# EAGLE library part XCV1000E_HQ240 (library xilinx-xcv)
xcv1000e_hq240 edit this description Auto generated by make-symbol-device-package-bsdl.ulp Rev. 26 Source: xcv1000e_hq240.bsd
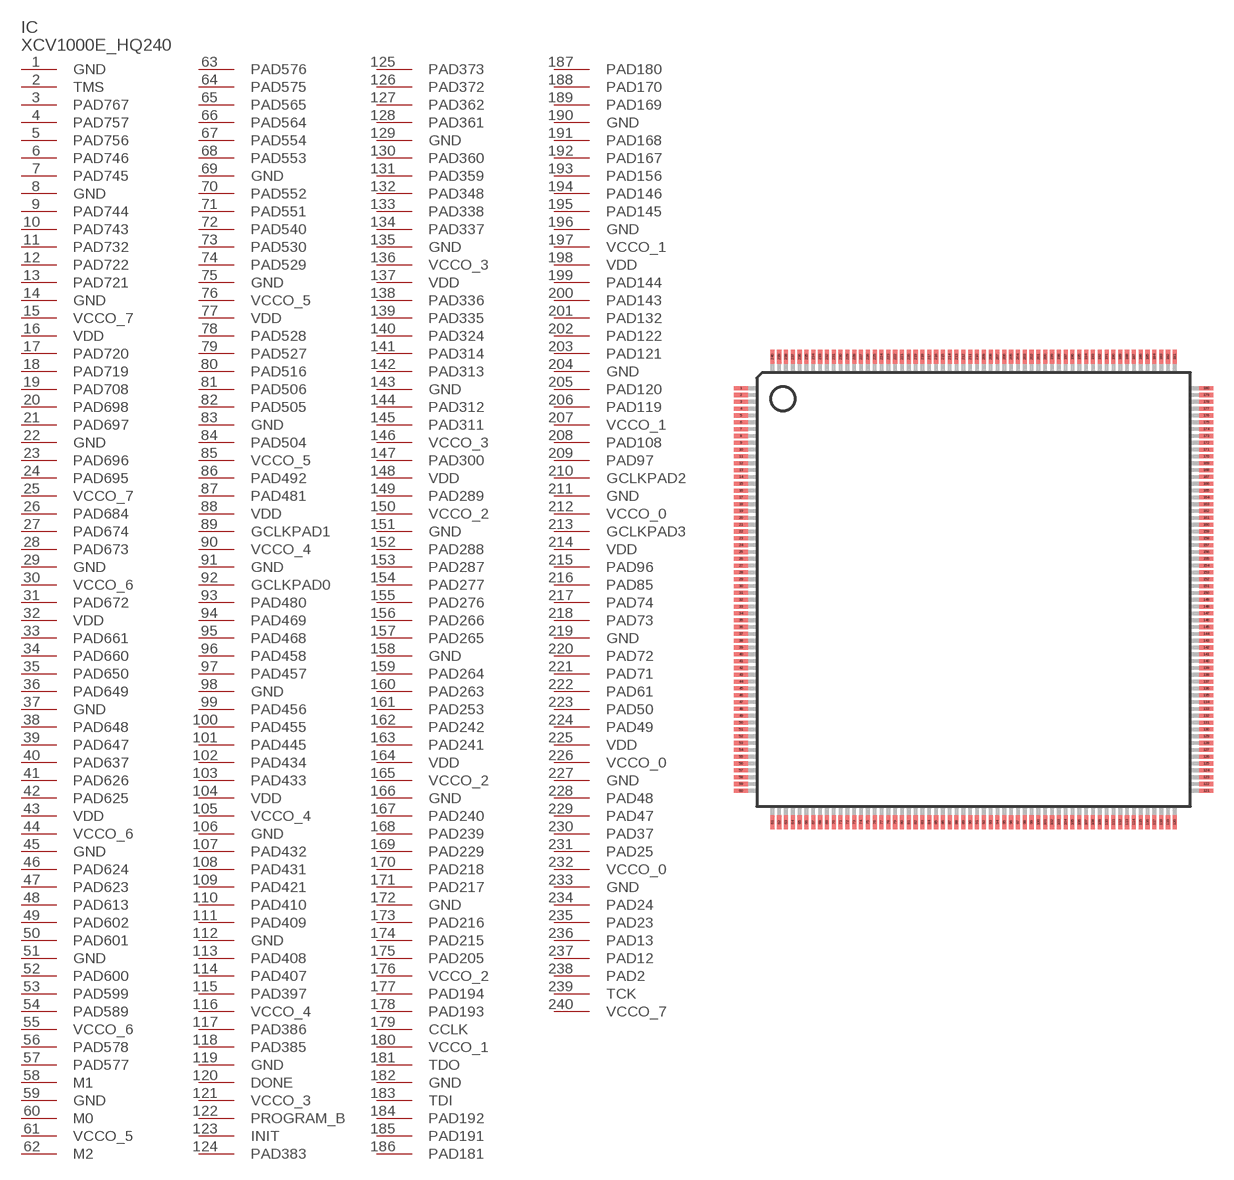
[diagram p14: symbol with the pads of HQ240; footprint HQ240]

Designator prefix IC

## XCV1000E_HQ240 (OC_FARNELL: unknown; OC_NEWARK: unknown)  [HQ240]
1  GND  pwr
2  TMS  in
3  PAD767
4  PAD757
5  PAD756
6  PAD746
7  PAD745
8  GND  pwr
9  PAD744
10  PAD743
11  PAD732
12  PAD722
13  PAD721
14  GND  pwr
15  VCCO_7  pwr
16  VDD  pwr
17  PAD720
18  PAD719
19  PAD708
20  PAD698
21  PAD697
22  GND  pwr
23  PAD696
24  PAD695
25  VCCO_7  pwr
26  PAD684
27  PAD674
28  PAD673
29  GND  pwr
30  VCCO_6  pwr
31  PAD672
32  VDD  pwr
33  PAD661
34  PAD660
35  PAD650
36  PAD649
37  GND  pwr
38  PAD648
39  PAD647
40  PAD637
41  PAD626
42  PAD625
43  VDD  pwr
44  VCCO_6  pwr
45  GND  pwr
46  PAD624
47  PAD623
48  PAD613
49  PAD602
50  PAD601
51  GND  pwr
52  PAD600
53  PAD599
54  PAD589
55  VCCO_6  pwr
56  PAD578
57  PAD577
58  M1  in
59  GND  pwr
60  M0  in
61  VCCO_5  pwr
62  M2  in
63  PAD576
64  PAD575
65  PAD565
66  PAD564
67  PAD554
68  PAD553
69  GND  pwr
70  PAD552
71  PAD551
72  PAD540
73  PAD530
74  PAD529
75  GND  pwr
76  VCCO_5  pwr
77  VDD  pwr
78  PAD528
79  PAD527
80  PAD516
81  PAD506
82  PAD505
83  GND  pwr
84  PAD504
85  VCCO_5  pwr
86  PAD492
87  PAD481
88  VDD  pwr
89  GCLKPAD1  in
90  VCCO_4  pwr
91  GND  pwr
92  GCLKPAD0  in
93  PAD480
94  PAD469
95  PAD468
96  PAD458
97  PAD457
98  GND  pwr
99  PAD456
100  PAD455
101  PAD445
102  PAD434
103  PAD433
104  VDD  pwr
105  VCCO_4  pwr
106  GND  pwr
107  PAD432
108  PAD431
109  PAD421
110  PAD410
111  PAD409
112  GND  pwr
113  PAD408
114  PAD407
115  PAD397
116  VCCO_4  pwr
117  PAD386
118  PAD385
119  GND  pwr
120  DONE
121  VCCO_3  pwr
122  PROGRAM_B  in
123  INIT
124  PAD383
125  PAD373
126  PAD372
127  PAD362
128  PAD361
129  GND  pwr
130  PAD360
131  PAD359
132  PAD348
133  PAD338
134  PAD337
135  GND  pwr
136  VCCO_3  pwr
137  VDD  pwr
138  PAD336
139  PAD335
140  PAD324
141  PAD314
142  PAD313
143  GND  pwr
144  PAD312
145  PAD311
146  VCCO_3  pwr
147  PAD300
148  VDD  pwr
149  PAD289
150  VCCO_2  pwr
151  GND  pwr
152  PAD288
153  PAD287
154  PAD277
155  PAD276
156  PAD266
157  PAD265
158  GND  pwr
159  PAD264
160  PAD263
161  PAD253
162  PAD242
163  PAD241
164  VDD  pwr
165  VCCO_2  pwr
166  GND  pwr
167  PAD240
168  PAD239
169  PAD229
170  PAD218
171  PAD217
172  GND  pwr
173  PAD216
174  PAD215
175  PAD205
176  VCCO_2  pwr
177  PAD194
178  PAD193
179  CCLK
180  VCCO_1  pwr
181  TDO  out
182  GND  pwr
183  TDI  in
184  PAD192
185  PAD191
186  PAD181
187  PAD180
188  PAD170
189  PAD169
190  GND  pwr
191  PAD168
192  PAD167
193  PAD156
194  PAD146
195  PAD145
196  GND  pwr
197  VCCO_1  pwr
198  VDD  pwr
199  PAD144
200  PAD143
201  PAD132
202  PAD122
203  PAD121
204  GND  pwr
205  PAD120
206  PAD119
207  VCCO_1  pwr
208  PAD108
209  PAD97
210  GCLKPAD2  in
211  GND  pwr
212  VCCO_0  pwr
213  GCLKPAD3  in
214  VDD  pwr
215  PAD96
216  PAD85
217  PAD74
218  PAD73
219  GND  pwr
220  PAD72
221  PAD71
222  PAD61
223  PAD50
224  PAD49
225  VDD  pwr
226  VCCO_0  pwr
227  GND  pwr
228  PAD48
229  PAD47
230  PAD37
231  PAD25
232  VCCO_0  pwr
233  GND  pwr
234  PAD24
235  PAD23
236  PAD13
237  PAD12
238  PAD2
239  TCK  in
240  VCCO_7  pwr

## Footprint HQ240 (pad centres in mm)
HQ240 Auto generated by make-symbol-device-package-bsdl.ulp Rev. 26
smd 1 x 0.3: 1 -17.05,14.75; 2 -17.05,14.25; 3 -17.05,13.75; 4 -17.05,13.25; 5 -17.05,12.75; 6 -17.05,12.25; 7 -17.05,11.75; 8 -17.05,11.25; 9 -17.05,10.75; 10 -17.05,10.25; 11 -17.05,9.75; 12 -17.05,9.25; 13 -17.05,8.75; 14 -17.05,8.25; 15 -17.05,7.75; 16 -17.05,7.25; 17 -17.05,6.75; 18 -17.05,6.25; 19 -17.05,5.75; 20 -17.05,5.25; 21 -17.05,4.75; 22 -17.05,4.25; 23 -17.05,3.75; 24 -17.05,3.25; 25 -17.05,2.75; 26 -17.05,2.25; 27 -17.05,1.75; 28 -17.05,1.25; 29 -17.05,0.75; 30 -17.05,0.25; 31 -17.05,-0.25; 32 -17.05,-0.75; 33 -17.05,-1.25; 34 -17.05,-1.75; 35 -17.05,-2.25; 36 -17.05,-2.75; 37 -17.05,-3.25; 38 -17.05,-3.75; 39 -17.05,-4.25; 40 -17.05,-4.75; 41 -17.05,-5.25; 42 -17.05,-5.75; 43 -17.05,-6.25; 44 -17.05,-6.75; 45 -17.05,-7.25; 46 -17.05,-7.75; 47 -17.05,-8.25; 48 -17.05,-8.75; 49 -17.05,-9.25; 50 -17.05,-9.75; 51 -17.05,-10.25; 52 -17.05,-10.75; 53 -17.05,-11.25; 54 -17.05,-11.75; 55 -17.05,-12.25; 56 -17.05,-12.75; 57 -17.05,-13.25; 58 -17.05,-13.75; 59 -17.05,-14.25; 60 -17.05,-14.75; 121 17.05,-14.75; 122 17.05,-14.25; 123 17.05,-13.75; 124 17.05,-13.25; 125 17.05,-12.75; 126 17.05,-12.25; 127 17.05,-11.75; 128 17.05,-11.25; 129 17.05,-10.75; 130 17.05,-10.25; 131 17.05,-9.75; 132 17.05,-9.25; 133 17.05,-8.75; 134 17.05,-8.25; 135 17.05,-7.75; 136 17.05,-7.25; 137 17.05,-6.75; 138 17.05,-6.25; 139 17.05,-5.75; 140 17.05,-5.25; 141 17.05,-4.75; 142 17.05,-4.25; 143 17.05,-3.75; 144 17.05,-3.25; 145 17.05,-2.75; 146 17.05,-2.25; 147 17.05,-1.75; 148 17.05,-1.25; 149 17.05,-0.75; 150 17.05,-0.25; 151 17.05,0.25; 152 17.05,0.75; 153 17.05,1.25; 154 17.05,1.75; 155 17.05,2.25; 156 17.05,2.75; 157 17.05,3.25; 158 17.05,3.75; 159 17.05,4.25; 160 17.05,4.75; 161 17.05,5.25; 162 17.05,5.75; 163 17.05,6.25; 164 17.05,6.75; 165 17.05,7.25; 166 17.05,7.75; 167 17.05,8.25; 168 17.05,8.75; 169 17.05,9.25; 170 17.05,9.75; 171 17.05,10.25; 172 17.05,10.75; 173 17.05,11.25; 174 17.05,11.75; 175 17.05,12.25; 176 17.05,12.75; 177 17.05,13.25; 178 17.05,13.75; 179 17.05,14.25; 180 17.05,14.75
smd 0.3 x 1: 61 -14.75,-17.05; 62 -14.25,-17.05; 63 -13.75,-17.05; 64 -13.25,-17.05; 65 -12.75,-17.05; 66 -12.25,-17.05; 67 -11.75,-17.05; 68 -11.25,-17.05; 69 -10.75,-17.05; 70 -10.25,-17.05; 71 -9.75,-17.05; 72 -9.25,-17.05; 73 -8.75,-17.05; 74 -8.25,-17.05; 75 -7.75,-17.05; 76 -7.25,-17.05; 77 -6.75,-17.05; 78 -6.25,-17.05; 79 -5.75,-17.05; 80 -5.25,-17.05; 81 -4.75,-17.05; 82 -4.25,-17.05; 83 -3.75,-17.05; 84 -3.25,-17.05; 85 -2.75,-17.05; 86 -2.25,-17.05; 87 -1.75,-17.05; 88 -1.25,-17.05; 89 -0.75,-17.05; 90 -0.25,-17.05; 91 0.25,-17.05; 92 0.75,-17.05; 93 1.25,-17.05; 94 1.75,-17.05; 95 2.25,-17.05; 96 2.75,-17.05; 97 3.25,-17.05; 98 3.75,-17.05; 99 4.25,-17.05; 100 4.75,-17.05; 101 5.25,-17.05; 102 5.75,-17.05; 103 6.25,-17.05; 104 6.75,-17.05; 105 7.25,-17.05; 106 7.75,-17.05; 107 8.25,-17.05; 108 8.75,-17.05; 109 9.25,-17.05; 110 9.75,-17.05; 111 10.25,-17.05; 112 10.75,-17.05; 113 11.25,-17.05; 114 11.75,-17.05; 115 12.25,-17.05; 116 12.75,-17.05; 117 13.25,-17.05; 118 13.75,-17.05; 119 14.25,-17.05; 120 14.75,-17.05; 181 14.75,17.05; 182 14.25,17.05; 183 13.75,17.05; 184 13.25,17.05; 185 12.75,17.05; 186 12.25,17.05; 187 11.75,17.05; 188 11.25,17.05; 189 10.75,17.05; 190 10.25,17.05; 191 9.75,17.05; 192 9.25,17.05; 193 8.75,17.05; 194 8.25,17.05; 195 7.75,17.05; 196 7.25,17.05; 197 6.75,17.05; 198 6.25,17.05; 199 5.75,17.05; 200 5.25,17.05; 201 4.75,17.05; 202 4.25,17.05; 203 3.75,17.05; 204 3.25,17.05; 205 2.75,17.05; 206 2.25,17.05; 207 1.75,17.05; 208 1.25,17.05; 209 0.75,17.05; 210 0.25,17.05; 211 -0.25,17.05; 212 -0.75,17.05; 213 -1.25,17.05; 214 -1.75,17.05; 215 -2.25,17.05; 216 -2.75,17.05; 217 -3.25,17.05; 218 -3.75,17.05; 219 -4.25,17.05; 220 -4.75,17.05; 221 -5.25,17.05; 222 -5.75,17.05; 223 -6.25,17.05; 224 -6.75,17.05; 225 -7.25,17.05; 226 -7.75,17.05; 227 -8.25,17.05; 228 -8.75,17.05; 229 -9.25,17.05; 230 -9.75,17.05; 231 -10.25,17.05; 232 -10.75,17.05; 233 -11.25,17.05; 234 -11.75,17.05; 235 -12.25,17.05; 236 -12.75,17.05; 237 -13.25,17.05; 238 -13.75,17.05; 239 -14.25,17.05; 240 -14.75,17.05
